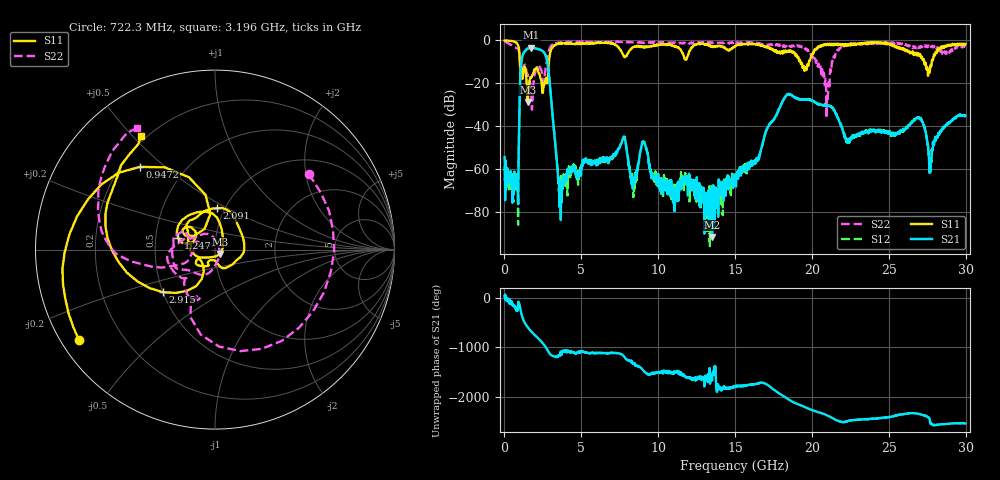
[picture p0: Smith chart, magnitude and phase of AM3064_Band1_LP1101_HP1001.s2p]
# Hz S DB R 50.0
!freq dBS11 angS11 dBS21 angS21 dBS12 angS12 dBS22 angS22
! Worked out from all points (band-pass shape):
!   1600 points, 10 MHz to 29.98 GHz, reference 50 ohm
!   highest |S21| = -3.45 dB at 1.753 GHz (marker M1); lowest = -91.6 dB at 13.51 GHz (marker M2)
!   |S21| within 3 dB of the highest: 1.207 GHz to 2.64 GHz (1.434 GHz wide, 74.5 % of centre)
!   lowest |S11| = -28.6 dB at 1.51 GHz (marker M3), VSWR 1.08, Z = 52.8 - j2.59 ohm
!   |S11| at or under -10 dB: 1.002 GHz to 2.893 GHz (1.891 GHz wide, 97.1 % of centre); 19.25 GHz to 19.81 GHz (557.8 MHz wide, 2.86 % of centre); 27.3 GHz to 27.8 GHz (496.9 MHz wide, 1.8 % of centre)
!   |S22| runs from -36.3 to -0.4 dB; largest |S21 - S12| = 0.0088
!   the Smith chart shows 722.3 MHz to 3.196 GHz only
!   S11 on the Smith chart (normalised r, x): 722.3 MHz: 0.05, -0.30; 947.2 MHz: 0.28, +0.41; 1.247 GHz: 0.65, +0.09; 2.091 GHz: 0.92, +0.45; 2.915 GHz: 0.50, -0.28; 3.196 GHz: 0.18, +0.53
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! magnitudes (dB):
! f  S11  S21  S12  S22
! 10 MHz  -0.1  -54.4  -58.4  -0.4
! 722.3 MHz  -0.8  -66.4  -68.9  -3.5
! 947.2 MHz  -4.1  -43.7  -43.6  -5.3
! 1.247 GHz  -13.3  -5.9  -5.8  -12.2
! 1.51 GHz  -28.6  -3.8  -3.8  -15.8
! 1.753 GHz  -17.3  -3.5  -3.4  -26.6
! 2.091 GHz  -12.7  -3.9  -3.9  -12.3
! 2.915 GHz  -8.5  -17.4  -17.4  -4.3
! 3.196 GHz  -2.5  -40.0  -39.9  -1.9
! 3.646 GHz  -1.4  -76.3  -67.2  -0.9
! 5.015 GHz  -1.5  -57.9  -59.4  -0.7
! 7.751 GHz  -7.3  -45.1  -45.3  -0.8
! 10 GHz  -2.1  -62.2  -67.3  -1.0
! 13.51 GHz  -2.7  -91.6  -78.6  -1.1
! 15 GHz  -2.7  -63.6  -62.6  -1.4
! 19.99 GHz  -7.6  -27.9  -27.9  -6.9
! 20.98 GHz  -1.8  -30.5  -30.2  -25.9
! 21.9 GHz  -2.2  -40.1  -39.2  -2.8
! 25 GHz  -1.4  -42.6  -43.1  -1.2
! 27 GHz  -7.0  -36.6  -36.1  -3.2
! 27.71 GHz  -11.5  -58.8  -57.1  -2.6
! 29.98 GHz  -1.7  -35.1  -35.1  -2.8
